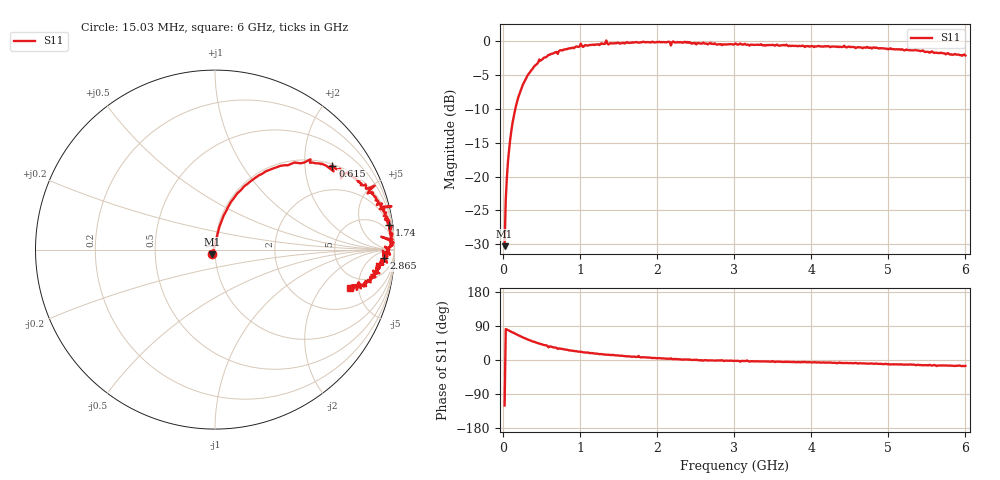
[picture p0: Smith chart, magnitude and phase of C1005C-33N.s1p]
!	Network	Analyzer	HP8753E.07.74:	Oct	30	2002	Serial	No.	JP38451487
!	Hewlett-Packard
!	7	Sep	2009	9:04:20
!	Frequency	S11
#	HZ	S	RI	R	50
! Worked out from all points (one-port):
!   400 points, 15.03 MHz to 6 GHz, reference 50 ohm
!   lowest |S11| = -30.3 dB at 15.03 MHz (marker M1), VSWR 1.06, Z = 48.4 - j2.57 ohm
!   |S11| at or under -10 dB: start of sweep to 154.4 MHz
!   S11 on the Smith chart (normalised r, x): 15.03 MHz: 0.97, -0.05; 615 MHz: 1.05, +2.76; 1.74 GHz: 2, +14; 2.865 GHz: 20, -17; 6 GHz: 3.65, -4.02
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1.502992e7  -0.0153 -0.0265
3.002985e7  0.00991 0.0671
6.00297e7  0.0253 0.129
1.050295e8  0.0617 0.214
1.650292e8  0.124 0.313
3.150284e8  0.329 0.454
6.150269e8  0.654 0.467
7.050265e8  0.701 0.395
7.650262e8  0.743 0.419
1.005025e9  0.89 0.356
1.035025e9  0.85 0.313
1.320023e9  0.926 0.239
1.335023e9  0.983 0.241
1.365023e9  0.918 0.226
1.515022e9  0.94 0.187
1.740021e9  0.97 0.137
1.755021e9  0.957 0.184
1.785021e9  0.974 0.114
2.145019e9  0.989 0.0564
2.175019e9  0.926 0.0717
2.205019e9  0.995 0.0383
2.265019e9  0.985 0.0393
2.865016e9  0.942 -0.0477
3.015015e9  0.961 -0.0376
3.765011e9  0.919 -0.0815
4.515007e9  0.899 -0.126
5.265004e9  0.84 -0.18
6e9  0.754 -0.213
